[IBIS ver]   3.2
[File name]   sprm205b.ibs
[File Rev]   1.4
[Date]   Mar 27, 2006
[Disclaimer]   Please be aware that in the absence of a written agreement
|   Texas Instruments(TI) assumes no liability for:
|   (1) The accuracy of the IBIS models provided to your company
|   (2) The proper functioning of these Models in your design
|   or for any resulting applications
|   (3) Infringement of patents, copyrights or intellectual
|   property rights resulting from your use of these
|   models.
|   TI provides IBIS Models as a service to our customers and
|   therefore reserves the right to limit distribution of the
|   Models.
|   The information is subject to change without
|   notice.
[Copyright]   Property of Texas Instruments Incorporated.
|   Unauthorized reproduction and/or distribution is strictly.
|   prohibited.
|   This product is protected under copyright law and trade
|   secret law as an unpublished work.
|   Created 2003,(C) Copyright 1999-2003,
|   Texas Instruments Incorporated., All Rights Reserved.
|   These commodities are under the U.S. Government
|   distribution license control. As such,they are not to be
|   re-exported without the prior approval of the U.S.
|   Department of Commerce.
[Notes]
|   Some IV curves contain Non monotonic data
|   points.
|   Component C6455
[Component]   C6455
[Manufacturer]   Texas Instruments.
[Package]
| variable   typ   min   max
R_pkg   5.92E-01   2.06E-01   1.13E+00
L_pkg   2.81E-09   3.46E-10   4.56E-09
C_pkg   1.31E-12   8.61E-13   2.06E-12
[Pin]   signal_name   model_name   R_pin   L_pin   C_pin
AG4   VTXD3/FSX1/GP[11] BT3350DTHYPDFZSCP18   6.09E-01   2.80E-09   1.37E-12
AE5   VTXD2/FSR1/GP[10] BT3350DTHYPDFZSCP18   7.48E-01   2.34E-09   1.40E-12
AG5   VTXD1/DX1/GP[9]   BT3350DTHYPDFZSCP18   8.37E-01   2.90E-09   1.51E-12
AH5   VTXD0/DR1/GP[8]   BT3350DTHYPDFZSCP18   5.24E-01   3.12E-09   1.35E-12
AG6   VSCRUNz/CLKX0   BT3325ETHYPUFZSCP18   6.27E-01   2.86E-09   1.41E-12
AJ3   VRXD3/FSX0   BT3350DTHYPDFZSCP18   5.12E-01   3.46E-09   1.32E-12
AH3   VRXD2/FSR0   BT3350DTHYPDFZSCP18   8.46E-01   3.26E-09   1.65E-12
AF6   VRXD1/DX0   BT3350DTHYPDFZSCP18   7.73E-01   2.43E-09   1.47E-12
AJ5   VRXD0/DR0   BT3350DTHYPDFZSCP18   7.02E-01   3.32E-09   1.12E-12
AG1   VCLK/CLKR0   BT3325ETHYPUFZSCP18   5.49E-01   3.71E-09   1.40E-12
K3   UXSOC/MCOL/GMCOL  BT3350CTHYPDFZP18   3.31E-01   2.22E-09   1.04E-12
J5   UXENBz/MTXEN/RMTXEN BT3350CTHYPUFZP18   4.33E-01   1.80E-09   1.10E-12
N5   UXDATA7/GMTXD7   BT3350CTHYPUFZP18   4.15E-01   1.72E-09   1.08E-12
M3   UXDATA6/GMTXD6   BT3350CTHYPUFZP18   6.89E-01   2.16E-09   1.45E-12
L5   UXDATA5/GMTXD5   BT3350CTHYPUFZP18   6.34E-01   1.81E-09   1.41E-12
L3   UXDATA4/GMTXD4   BT3350CTHYPUFZP18   4.95E-01   2.20E-09   1.22E-12
K4   UXDATA3/MTXD3/GMTXD3 BT3350CTHYPUFZP18  6.82E-01   2.13E-09   1.38E-12
M4   UXDATA2/MTXD2/GMTXD2 BT3350CTHYPUFZP18  4.56E-01   1.96E-09   1.11E-12
L4   UXDATA1/MTXD1/RMTXD1 BT3350CTHYPUFZP18  2.86E-01   1.93E-09   1.06E-12
M1   UXDATA0/MTXD0/RMTXD0 BT3350CTHYPUFZP18  5.78E-01   2.81E-09   1.38E-12
N4   UXCLK/MTCLK/REFCLK BT3350DTHYPUFZSCP18  2.83E-01   1.84E-09   9.18E-13
K5   UXCLAV/GMTCLK   BT3350DTHYPDFZSCP18   4.28E-01   1.79E-09   1.14E-12
M5   UXADDR4/GMDCLK   BT3350CTHYPUFZP18   2.46E-01   1.67E-09   9.84E-13
N3   UXADDR3/GMDIO   BT3350CTHYPUFZP18   6.98E-01   2.32E-09   1.47E-12
P5   UXADDR2/PCBE3z   BPCI66RCGPUFZP18   4.09E-01   1.70E-09   1.09E-12
R3   UXADDR1/PIDSEL   BPCI66RCGPUFZP18   3.11E-01   2.12E-09   1.04E-12
P4   UXADDR0/PTRDYz   BPCI66RCGPUFZP18   6.39E-01   1.91E-09   1.40E-12
H4   URSOC/MRXER/RMRXER   BT3350CTHYPUFZP18  2.98E-01   1.99E-09   1.07E-12
H5   URENBz/MRXDV   BT3350CTHYPUFZP18   6.52E-01   1.96E-09   1.34E-12
M2   URDATA7/MRXD7   BT3350CTHYPUFZP18   3.58E-01   2.56E-09   1.02E-12
H2   URDATA6/MRXD6   BT3350CTHYPUFZP18   7.86E-01   2.83E-09   1.52E-12
L2   URDATA5/MRXD5   BT3350CTHYPUFZP18   7.58E-01   2.79E-09   1.61E-12
L1   URDATA4/MRXD4   BT3350CTHYPUFZP18   5.76E-01   2.73E-09   1.37E-12
J3   URDATA3/MRXD3   BT3350CTHYPUFZP18   5.17E-01   2.35E-09   1.24E-12
J1   URDATA2/MRXD2   BT3350CTHYPUFZP18   4.37E-01   2.85E-09   1.35E-12
H3   URDATA1/MRXD1/RMRXD1 BT3350CTHYPUFZP18  5.29E-01   2.45E-09   1.32E-12
J2   URDATA0/MRXD0/RMRXD0 BT3350CTHYPUFZP18  7.85E-01   2.80E-09   1.57E-12
H1   URCLK/MRCLK/GMRCLK   BT3350CTHYPUFZP18  4.59E-01   3.04E-09   1.26E-12
J4   URCLAV/MCRS/RMCRSDV  BT3350CTHYPDFZP18  6.78E-01   2.16E-09   1.45E-12
P1   URADDR4/PCBE0z/GP[2] BPCI66RCGPUFZP18   7.61E-01   2.71E-09   1.51E-12
P2   URADDR3/PREQz/GP[15] BPCI66RCGPUFZP18   5.35E-01   2.52E-09   1.27E-12
P3   URADDR2/PINTAz/GP14  BPCI66RCGPUFZP18   3.31E-01   2.20E-09   1.08E-12
R5   URADDR1/PRSTz/GP[13] BPCI66RCGPUFZP18   2.21E-01   1.50E-09   9.28E-13
R4   URADDR0/PGNTz/GP[12] BPCI66RCGPUFZP18   6.52E-01   1.98E-09   1.31E-12
AH7   TRST   IT33THYPDFZP18   4.68E-01   2.81E-09   1.20E-12
AG7   TOUTL1   BT3350CTHYPDFZP18   8.09E-01   2.65E-09   1.68E-12
AF8   TOUTL0   BT3350CTHYPDFZP18   7.76E-01   2.33E-09   1.43E-12
AJ10   TMS   IT33THYPUFZP18   8.57E-01   2.81E-09   1.63E-12
AJ6   TINPL1   BT3350CTHYPDFZP18   4.92E-01   2.86E-09   1.02E-12
AH6   TINPL0   BT3350CTHYPDFZP18   8.68E-01   3.06E-09   1.72E-12
AH8   TDO   BT3350DTHYPUFZSCP18   5.88E-01   2.38E-09   1.08E-12
AH9   TDI   IT33THYPUFZP18   6.08E-01   2.69E-09   1.30E-12
AJ9   TCK   IT33THYPUFZP18   8.56E-01   3.03E-09   1.59E-12
AJ13   SYSCLK3/GP[1]   BT3325ETHYPDFZSCP18   6.03E-01   2.77E-09   1.32E-12
AF26   SDA   BI2CTFZP18   8.57E-01   3.03E-09   1.71E-12
AG26   SCL   BI2CTFZP18   6.79E-01   3.07E-09   1.37E-12
AF15   RIOCLK   ICLKRX18G   5.07E-01   2.13E-09   1.25E-12
AG15   RIOCLKz   ICLKRX18G   7.35E-01   2.18E-09   1.43E-12
D3   RGTXCTL   BHSTLDVG   8.45E-01   2.76E-09   1.50E-12
D4   RGMTCLK   BHSTLDVG   6.15E-01   2.80E-09   1.29E-12
A2   RGMTD3   BHSTLDVG   5.94E-01   3.66E-09   1.40E-12
C3   RGMTD2   BHSTLDVG   8.89E-01   3.06E-09   1.64E-12
B3   RGMTD1   BHSTLDVG   9.28E-01   3.30E-09   1.78E-12
A3   RGMTD0   BHSTLDVG   7.46E-01   3.55E-09   1.43E-12
C2   RGMRXCTL   BHSTLDVG   4.83E-01   3.03E-09   1.27E-12
E3   RGMRCLK   BHSTLDVG   7.50E-01   2.59E-09   1.49E-12
C1   RGMRXD3   BHSTLDVG   8.67E-01   3.27E-09   1.63E-12
E4   RGMRXD2   BHSTLDVG   5.25E-01   2.45E-09   1.28E-12
E2   RGMRXD1   BHSTLDVG   4.36E-01   2.95E-09   1.29E-12
E1   RGMRXD0   BHSTLDVG   6.31E-01   3.09E-09   1.10E-12
A4   RGMDIO   BHSTLDVG   7.36E-01   3.49E-09   1.07E-12
B4   RGMDCLK   BHSTLDVG   9.25E-01   3.27E-09   1.59E-12
C4   RGREFCLK   BHSTLDVG   4.98E-01   2.98E-09   1.20E-12
AG14   RESETz   IT33THYP18   5.06E-01   2.06E-09   1.15E-12
AE14   RESETSTATz   BT3350CTHYPUFZP18   6.38E-01   1.67E-09   1.31E-12
Y29   PCI_EN   BT3350CTHYPDFZP18   9.60E-01   3.24E-09   1.91E-12
AH4   NMI   BT3350CTHYPDFZP18   9.04E-01   3.32E-09   1.67E-12
T5   HRWz/PCBE2z   BPCI66RCGPUFZP18   2.43E-01   1.60E-09   1.01E-12
T4   HRDYz/PIRDYz   BPCI66RCGPUFZP18   6.49E-01   2.01E-09   1.30E-12
U3   HINTz/PFRAMEz   BPCI66RCGPUFZP18   3.23E-01   2.16E-09   1.14E-12
V3   HHWIL/PCLK   BPCI66RCGPUFZP18   5.12E-01   2.31E-09   1.28E-12
U1   HDS2z/PCBE1z   BPCI66RCGPUFZP18   5.78E-01   2.75E-09   1.14E-12
U2   HDS1z/PSERRz   BPCI66RCGPUFZP18   7.38E-01   2.52E-09   1.46E-12
AA3   HD31/AD31   BPCI66RCGPUFZP18   3.58E-01   2.34E-09   1.14E-12
AA5   HD30/AD30   BPCI66RCGPUFZP18   6.55E-01   2.01E-09   1.37E-12
AC4   HD29/AD29   BPCI66RCGPUFZP18   3.31E-01   2.22E-09   1.11E-12
AA4   HD28/AD28   BPCI66RCGPUFZP18   4.88E-01   2.19E-09   1.08E-12
AC5   HD27/AD27   BPCI66RCGPUFZP18   6.86E-01   2.25E-09   1.38E-12
Y1   HD26/AD26   BPCI66RCGPUFZP18   4.37E-01   2.86E-09   1.30E-12
AD2   HD25/AD25   BPCI66RCGPUFZP18   6.04E-01   2.89E-09   1.50E-12
W1   HD24/AD24   BPCI66RCGPUFZP18   8.01E-01   2.91E-09   1.55E-12
AC3   HD23/AD23   BPCI66RCGPUFZP18   7.58E-01   2.69E-09   1.33E-12
AE1   HD22/AD22   BPCI66RCGPUFZP18   6.55E-01   3.17E-09   1.58E-12
AD1   HD21/AD21   BPCI66RCGPUFZP18   4.66E-01   3.11E-09   1.31E-12
W2   HD20/AD20   BPCI66RCGPUFZP18   3.62E-01   2.14E-09   1.16E-12
AC1   HD19/AD19   BPCI66RCGPUFZP18   8.42E-01   3.24E-09   1.66E-12
Y2   HD18/AD18   BPCI66RCGPUFZP18   5.80E-01   2.76E-09   1.37E-12
AB1   HD17/AD17   BPCI66RCGPUFZP18   4.42E-01   2.91E-09   1.42E-12
Y3   HD16/AD16   BPCI66RCGPUFZP18   7.19E-01   2.42E-09   1.39E-12
AB2   HD15/AD15   BPCI66RCGPUFZP18   5.75E-01   2.77E-09   1.38E-12
W4   HD14/AD14   BPCI66RCGPUFZP18   6.64E-01   2.06E-09   1.39E-12
AC2   HD13/AD13   BPCI66RCGPUFZP18   6.09E-01   2.99E-09   1.42E-12
V4   HD12/AD12   BPCI66RCGPUFZP18   6.63E-01   2.02E-09   1.46E-12
AF3   HD11/AD11   BPCI66RCGPUFZP18   8.21E-01   2.98E-09   1.63E-12
AE3   HD10/AD10   BPCI66RCGPUFZP18   5.92E-01   2.89E-09   1.46E-12
AB3   HD9/AD9   BPCI66RCGPUFZP18   7.51E-01   2.70E-09   1.51E-12
W5   HD8/AD8   BPCI66RCGPUFZP18   2.56E-01   1.70E-09   1.02E-12
AB4   HD7/AD7   BPCI66RCGPUFZP18   3.35E-01   2.26E-09   1.15E-12
Y4   HD6/AD6   BPCI66RCGPUFZP18   4.92E-01   2.22E-09   1.27E-12
AD3   HD5/AD5   BPCI66RCGPUFZP18   7.69E-01   2.75E-09   1.55E-12
Y5   HD4/AD4   BPCI66RCGPUFZP18   6.44E-01   1.93E-09   1.34E-12
AD4   HD3/AD3   BPCI66RCGPUFZP18   3.57E-01   2.45E-09   1.10E-12
W6   HD2/AD2   BPCI66RCGPUFZP18   5.81E-01   1.49E-09   1.29E-12
AB5   HD1/AD1   BPCI66RCGPUFZP18   4.60E-01   1.99E-09   1.21E-12
AE2   HD0/AD0   BPCI66RCGPUFZP18   8.34E-01   3.24E-09   1.63E-12
U6   HCSz/PPERRz   BPCI66RCGPUFZP18   2.06E-01   1.34E-09   8.91E-13
U4   HCNTL1/PDEVSELz   BPCI66RCGPUFZP18   4.64E-01   1.99E-09   1.20E-12
U5   HCNTL0/PSTOPz   BPCI66RCGPUFZP18   6.24E-01   1.79E-09   1.35E-12
T3   HASz/PPAR   BPCI66RCGPUFZP18   4.95E-01   2.25E-09   1.27E-12
AG2   GP[7]   BT3350DTHYPDFZSCP18   6.54E-01   3.32E-09   1.22E-12
AG3   GP[6]   BT3350DTHYPDFZSCP18   8.29E-01   3.14E-09   1.54E-12
AJ2   GP[5]   BT3350DTHYPDFZSCP18   7.00E-01   3.62E-09   1.55E-12
AH2   GP[4]   BT3350DTHYPDFZSCP18   5.15E-01   3.56E-09   1.32E-12
AE11   EMU1   BT3325ETHYPUFZSCP18   6.49E-01   1.74E-09   1.42E-12
AF7   EMU0   BT3325ETHYPUFZSCP18   5.81E-01   2.43E-09   1.23E-12
AE13   EMU18   BT3325ETHYPUFZSCP18   4.33E-01   1.56E-09   1.08E-12
AH10   EMU17   BT3325ETHYPUFZSCP18   5.89E-01   2.53E-09   1.32E-12
AE9   EMU15   BT3325ETHYPUFZSCP18   4.89E-01   1.94E-09   1.19E-12
AF13   EMU14   BT3325ETHYPUFZSCP18   7.13E-01   1.94E-09   1.31E-12
AD8   EMU13   BT3325ETHYPUFZSCP18   4.61E-01   1.70E-09   1.10E-12
AE10   EMU12   BT3325ETHYPUFZSCP18   4.69E-01   1.70E-09   1.11E-12
AH12   EMU16   BT3325ETHYPUFZSCP18   5.85E-01   2.50E-09   1.36E-12
AD12   EMU11   BT3325ETHYPUFZSCP18   4.10E-01   1.36E-09   1.01E-12
AD10   EMU10   BT3325ETHYPUFZSCP18   2.51E-01   1.42E-09   9.05E-13
AH13   EMU9   BT3325ETHYPUFZSCP18   3.95E-01   2.43E-09   1.19E-12
AF11   EMU8   BT3325ETHYPUFZSCP18   3.39E-01   1.96E-09   1.03E-12
AF12   EMU7   BT3325ETHYPUFZSCP18   3.19E-01   1.85E-09   9.89E-13
AG8   EMU6   BT3325ETHYPUFZSCP18   4.29E-01   2.55E-09   1.09E-12
AE12   EMU5   BT3325ETHYPUFZSCP18   6.73E-01   1.73E-09   1.31E-12
AF9   EMU4   BT3325ETHYPUFZSCP18   7.37E-01   2.16E-09   1.61E-12
AF10   EMU3   BT3325ETHYPUFZSCP18   7.24E-01   2.11E-09   1.43E-12
AG9   EMU2   BT3325ETHYPUFZSCP18   3.93E-01   2.36E-09   1.04E-12
AF5   CLKX1/GP[3]   BT3325ETHYPDFZSCP18   5.75E-01   2.45E-09   1.30E-12
AJ4   CLKS   BT3350CTHYPDFZP18   5.43E-01   3.41E-09   1.28E-12
AF4   CLKR1/GP[0]   BT3325ETHYPDFZSCP18   4.15E-01   2.53E-09   1.08E-12
G3   CLKIN2   IT33THYPDFZP18   5.43E-01   2.57E-09   9.68E-13
N28   CLKIN1   IT33THYPDFZP18   6.35E-01   2.69E-09   1.38E-12
B13   DSDWEz   BSSTL18GFZ   3.59E-01   2.46E-09   1.18E-12
C13   DSDRASz   BSSTL18GFZ   4.96E-01   2.18E-09   1.09E-12
E23   DSDDQS3   BSSTL18GFZ   3.31E-01   2.14E-09   1.04E-12
D23   DSDDQS3z   BSSTL18GFZ   5.26E-01   2.40E-09   1.19E-12
E20   DSDDQS2   BSSTL18GFZ   7.19E-01   2.12E-09   1.35E-12
D20   DSDDQS2z   BSSTL18GFZ   3.16E-01   2.01E-09   1.08E-12
E8   DSDDQS1   BSSTL18GFZ   5.55E-01   2.46E-09   1.20E-12
D8   DSDDQS1z   BSSTL18GFZ   3.91E-01   2.40E-09   1.08E-12
E11   DSDDQS0   BSSTL18GFZ   7.21E-01   2.10E-09   1.34E-12
D11   DSDDQS0z   BSSTL18GFZ   4.92E-01   2.23E-09   1.16E-12
C23   DSDDQM3   BSSTL18GFZ   7.78E-01   2.61E-09   1.47E-12
C20   DSDDQM2   BSSTL18GFZ   5.24E-01   2.35E-09   1.04E-12
C8   DSDDQM1   BSSTL18GFZ   8.23E-01   2.75E-09   1.58E-12
C11   DSDDQM0   BSSTL18GFZ   3.52E-01   2.28E-09   1.06E-12
F21   DSDDQGATE3   BSSTL18GFZ   2.22E-01   1.50E-09   1.03E-12
E21   DSDDQGATE2   BSSTL18GFZ   4.37E-01   1.80E-09   1.15E-12
B9   DSDDQGATE1   BSSTL18GFZ   5.56E-01   2.53E-09   1.09E-12
A9   DSDDQGATE0   BSSTL18GFZ   4.51E-01   3.00E-09   1.23E-12
D14   DSDCKE   BSSTL18GFZ   4.41E-01   1.88E-09   9.67E-13
D13   DSDCASz   BSSTL18GFZ   7.00E-01   2.09E-09   1.52E-12
A17   DEODT[1]   BSSTL18GFZ   5.57E-01   2.63E-09   1.08E-12
E16   DEODT[0]   BSSTL18GFZ   6.32E-01   1.50E-09   1.27E-12
B25   DED31   BSSTL18GFZ   6.19E-01   3.04E-09   1.50E-12
A25   DED30   BSSTL18GFZ   8.99E-01   3.42E-09   1.78E-12
B24   DED29   BSSTL18GFZ   6.02E-01   2.96E-09   1.33E-12
A24   DED28   BSSTL18GFZ   8.38E-01   2.95E-09   1.53E-12
D22   DED27   BSSTL18GFZ   2.92E-01   1.85E-09   1.07E-12
C22   DED26   BSSTL18GFZ   9.49E-01   2.59E-09   1.69E-12
B22   DED25   BSSTL18GFZ   5.68E-01   2.69E-09   1.45E-12
A22   DED24   BSSTL18GFZ   8.07E-01   2.44E-09   1.71E-12
D21   DED23   BSSTL18GFZ   7.04E-01   2.05E-09   1.47E-12
C21   DED22   BSSTL18GFZ   3.65E-01   2.38E-09   1.11E-12
B21   DED21   BSSTL18GFZ   9.23E-01   2.25E-09   1.74E-12
A21   DED20   BSSTL18GFZ   5.99E-01   2.82E-09   1.20E-12
D19   DED19   BSSTL18GFZ   7.00E-01   2.12E-09   1.47E-12
C19   DED18   BSSTL18GFZ   3.37E-01   2.21E-09   1.08E-12
A19   DED17   BSSTL18GFZ   9.35E-01   2.18E-09   1.76E-12
B19   DED16   BSSTL18GFZ   5.41E-01   2.48E-09   1.28E-12
C7   DED15   BSSTL18GFZ   5.66E-01   2.55E-09   1.33E-12
D7   DED14   BSSTL18GFZ   9.91E-01   2.78E-09   1.63E-12
A7   DED13   BSSTL18GFZ   4.73E-01   2.84E-09   1.29E-12
B7   DED12   BSSTL18GFZ   8.82E-01   3.15E-09   1.65E-12
F9   DED11   BSSTL18GFZ   4.47E-01   1.90E-09   1.15E-12
E9   DED10   BSSTL18GFZ   8.86E-01   2.18E-09   1.59E-12
D9   DED9   BSSTL18GFZ   3.32E-01   2.16E-09   9.59E-13
C9   DED8   BSSTL18GFZ   7.83E-01   2.64E-09   1.58E-12
D10   DED7   BSSTL18GFZ   7.11E-01   2.12E-09   1.47E-12
C10   DED6   BSSTL18GFZ   5.45E-01   2.29E-09   1.06E-12
B10   DED5   BSSTL18GFZ   9.48E-01   2.75E-09   1.69E-12
A10   DED4   BSSTL18GFZ   4.37E-01   2.82E-09   1.29E-12
D12   DED3   BSSTL18GFZ   6.89E-01   1.97E-09   1.40E-12
C12   DED2   BSSTL18GFZ   4.96E-01   2.18E-09   1.06E-12
B12   DED1   BSSTL18GFZ   7.89E-01   2.63E-09   1.57E-12
A12   DED0   BSSTL18GFZ   5.97E-01   2.80E-09   1.17E-12
B14   DDR2CLKOUTP   BSSTL18GFZ   8.23E-01   2.80E-09   1.52E-12
A14   DDR2CLKOUTN   BSSTL18GFZ   6.03E-01   2.82E-09   1.06E-12
B15   DEA13   BSSTL18GFZ   7.58E-01   2.40E-09   1.58E-12
A15   DEA12   BSSTL18GFZ   5.68E-01   2.69E-09   1.35E-12
A16   DEA11   BSSTL18GFZ   3.85E-01   2.51E-09   1.15E-12
B16   DEA10   BSSTL18GFZ   7.91E-01   2.45E-09   1.44E-12
C16   DEA9   BSSTL18GFZ   4.86E-01   2.11E-09   1.36E-12
D16   DEA8   BSSTL18GFZ   2.77E-01   1.84E-09   1.12E-12
B17   DEA7   BSSTL18GFZ   3.56E-01   2.32E-09   1.18E-12
C17   DEA6   BSSTL18GFZ   7.14E-01   2.33E-09   1.47E-12
D17   DEA5   BSSTL18GFZ   4.44E-01   1.89E-09   1.13E-12
E17   DEA4   BSSTL18GFZ   6.41E-01   1.65E-09   1.36E-12
A18   DEA3   BSSTL18GFZ   5.60E-01   2.58E-09   1.19E-12
B18   DEA2   BSSTL18GFZ   3.73E-01   2.45E-09   1.02E-12
C18   DEA1   BSSTL18GFZ   7.36E-01   2.41E-09   1.39E-12
D18   DEA0   BSSTL18GFZ   4.52E-01   1.89E-09   1.19E-12
E14   DCE0z   BSSTL18GFZ   6.49E-01   1.70E-09   1.23E-12
E15   DBA2   BSSTL18GFZ   2.38E-01   1.52E-09   9.14E-13
D15   DBA1   BSSTL18GFZ   6.83E-01   1.93E-09   1.44E-12
C15   DBA0   BSSTL18GFZ   4.95E-01   2.23E-09   1.11E-12
AB25   AAWEz/ASWEz   BT3350DTHYPUFZSCP18   7.69E-01   1.99E-09   1.65E-12
W25   AR/Wz   BT3350DTHYPUFZSCP18   3.14E-01   1.65E-09   9.87E-13
Y28   AAOEz/ASOEz   BT3350DTHYPUFZSCP18   8.31E-01   2.20E-09   1.72E-12
R29   AHOLDz   BT3350CTHYPUFZP18   9.46E-01   3.13E-09   1.81E-12
N26   AHOLDAz   BT3350CTHYPUFZP18   5.24E-01   2.00E-09   1.23E-12
F25   AED63   BT3350DTHYPUFZSCP18   7.89E-01   2.15E-09   1.36E-12
A27   AED62   BT3350DTHYPUFZSCP18   7.72E-01   3.71E-09   1.62E-12
C27   AED61   BT3350DTHYPUFZSCP18   9.51E-01   3.23E-09   1.70E-12
C28   AED60   BT3350DTHYPUFZSCP18   7.67E-01   3.66E-09   1.45E-12
E27   AED59   BT3350DTHYPUFZSCP18   4.68E-01   2.81E-09   1.26E-12
D28   AED58   BT3350DTHYPUFZSCP18   9.58E-01   3.21E-09   1.69E-12
D27   AED57   BT3350DTHYPUFZSCP18   6.67E-01   2.99E-09   1.30E-12
F27   AED56   BT3350DTHYPUFZSCP18   6.45E-01   2.81E-09   1.25E-12
G25   AED55   BT3350DTHYPUFZSCP18   5.37E-01   2.10E-09   1.23E-12
G26   AED54   BT3350DTHYPUFZSCP18   4.19E-01   2.36E-09   1.16E-12
A28   AED53   BT3350DTHYPUFZSCP18   6.54E-01   3.93E-09   1.43E-12
F28   AED52   BT3350DTHYPUFZSCP18   9.26E-01   3.02E-09   2.03E-12
B28   AED51   BT3350DTHYPUFZSCP18   1.04E+00   3.74E-09   1.95E-12
G27   AED50   BT3350DTHYPUFZSCP18   6.38E-01   2.73E-09   1.34E-12
B27   AED49   BT3350DTHYPUFZSCP18   5.58E-01   3.17E-09   1.43E-12
G28   AED48   BT3350DTHYPUFZSCP18   4.85E-01   2.82E-09   1.19E-12
H25   AED47   BT3350DTHYPUFZSCP18   7.81E-01   2.11E-09   1.46E-12
J26   AED46   BT3350DTHYPUFZSCP18   8.14E-01   2.33E-09   1.57E-12
H26   AED45   BT3350DTHYPUFZSCP18   5.78E-01   2.36E-09   9.76E-13
J27   AED44   BT3350DTHYPUFZSCP18   5.96E-01   2.46E-09   1.32E-12
H27   AED43   BT3350DTHYPUFZSCP18   4.51E-01   2.58E-09   1.04E-12
J28   AED42   BT3350DTHYPUFZSCP18   4.69E-01   2.75E-09   1.22E-12
C29   AED41   BT3350DTHYPUFZSCP18   1.13E+00   4.35E-09   2.00E-12
J29   AED40   BT3350DTHYPUFZSCP18   9.53E-01   3.20E-09   1.86E-12
D29   AED39   BT3350DTHYPUFZSCP18   8.22E-01   3.89E-09   1.64E-12
J25   AED38   BT3350DTHYPUFZSCP18   3.47E-01   1.87E-09   9.91E-13
F29   AED37   BT3350DTHYPUFZSCP18   1.02E+00   3.63E-09   1.81E-12
F26   AED36   BT3350DTHYPUFZSCP18   8.37E-01   2.44E-09   1.66E-12
G29   AED35   BT3350DTHYPUFZSCP18   7.03E-01   3.11E-09   1.43E-12
K28   AED34   BT3350DTHYPUFZSCP18   5.98E-01   2.38E-09   1.45E-12
K25   AED33   BT3350DTHYPUFZSCP18   4.94E-01   1.76E-09   1.18E-12
K27   AED32   BT3350DTHYPUFZSCP18   8.53E-01   2.56E-09   1.72E-12
AA27   AED31   BT3350DTHYPUFZSCP18   5.91E-01   2.40E-09   1.33E-12
AG29   AED30   BT3350DTHYPUFZSCP18   7.73E-01   3.53E-09   1.63E-12
AB29   AED29   BT3350DTHYPUFZSCP18   7.00E-01   3.16E-09   1.20E-12
AC27   AED28   BT3350DTHYPUFZSCP18   4.26E-01   2.49E-09   1.13E-12
AB28   AED27   BT3350DTHYPUFZSCP18   4.67E-01   2.64E-09   1.12E-12
AC26   AED26   BT3350DTHYPUFZSCP18   8.05E-01   2.21E-09   1.60E-12
AB27   AED25   BT3350DTHYPUFZSCP18   8.55E-01   2.52E-09   1.64E-12
AC25   AED24   BT3350DTHYPUFZSCP18   5.12E-01   1.92E-09   1.15E-12
AB26   AED23   BT3350DTHYPUFZSCP18   5.46E-01   2.14E-09   1.28E-12
AD28   AED22   BT3350DTHYPUFZSCP18   4.68E-01   2.73E-09   1.08E-12
AD29   AED21   BT3350DTHYPUFZSCP18   9.46E-01   3.09E-09   1.86E-12
AJ28   AED20   BT3350DTHYPUFZSCP18   1.03E+00   4.07E-09   1.99E-12
AF29   AED19   BT3350DTHYPUFZSCP18   5.92E-01   3.44E-09   1.38E-12
AH28   AED18   BT3350DTHYPUFZSCP18   7.85E-01   3.68E-09   1.24E-12
AE29   AED17   BT3350DTHYPUFZSCP18   7.43E-01   3.46E-09   1.30E-12
AG28   AED16   BT3350DTHYPUFZSCP18   1.01E+00   3.59E-09   1.91E-12
AF28   AED15   BT3350DTHYPUFZSCP18   7.10E-01   3.12E-09   1.36E-12
AH26   AED14   BT3350DTHYPUFZSCP18   5.35E-01   3.16E-09   1.25E-12
AE28   AED13   BT3350DTHYPUFZSCP18   9.42E-01   3.10E-09   1.71E-12
AE26   AED12   BT3350DTHYPUFZSCP18   8.60E-01   3.00E-09   1.59E-12
AD26   AED11   BT3350DTHYPUFZSCP18   3.97E-01   2.39E-09   1.10E-12
AF27   AED10   BT3350DTHYPUFZSCP18   5.31E-01   3.20E-09   1.14E-12
AG27   AED9   BT3350DTHYPUFZSCP18   9.16E-01   3.29E-09   1.87E-12
AD27   AED8   BT3350DTHYPUFZSCP18   5.75E-01   2.48E-09   1.27E-12
AE25   AED7   BT3350DTHYPUFZSCP18   5.96E-01   2.68E-09   1.20E-12
AJ27   AED6   BT3350DTHYPUFZSCP18   6.28E-01   3.87E-09   1.50E-12
AJ26   AED5   BT3350DTHYPUFZSCP18   9.46E-01   3.47E-09   1.88E-12
AE27   AED4   BT3350DTHYPUFZSCP18   6.54E-01   3.06E-09   1.02E-12
AG25   AED3   BT3350DTHYPUFZSCP18   4.92E-01   3.03E-09   1.26E-12
AH27   AED2   BT3350DTHYPUFZSCP18   7.32E-01   3.30E-09   1.46E-12
AF25   AED1   BT3350DTHYPUFZSCP18   6.26E-01   2.91E-09   1.20E-12
AD25   AED0   BT3350DTHYPUFZSCP18   7.53E-01   2.34E-09   1.47E-12
V29   AECLKOUT   BT3325ETHYPDFZSCP18   9.72E-01   3.21E-09   2.06E-12
N29   AECLKIN   BT3350CTHYPDFZP18   9.47E-01   3.14E-09   1.80E-12
T26   AEA2/CFGGP2   BT3350DTHYPDFZSCP18   5.04E-01   1.89E-09   1.17E-12
N25   AEA19/BOOTMODE3   BT3350DTHYPDFZSCP18   3.15E-01   1.66E-09   9.71E-13
L26   AEA18/BOOTMODE2   BT3350DTHYPDFZSCP18   5.31E-01   2.00E-09   1.31E-12
L25   AEA17/BOOTMODE1   BT3350DTHYPDFZSCP18   7.40E-01   1.80E-09   1.58E-12
P26   AEA16/BOOTMODE0   BT3350DTHYPDFZSCP18   5.34E-01   2.05E-09   1.34E-12
P27   AEA15/AECLKIN_SEL BT3350DTHYPDFZSCP18   4.13E-01   2.30E-09   1.12E-12
R25   AEA14/HPI_WIDTH   BT3350DTHYPDFZSCP18   4.42E-01   1.39E-09   1.14E-12
R27   AEA13/LENDIAN   BT3350DTHYPDFZSCP18   3.97E-01   2.24E-09   1.17E-12
R28   AEA12/UTOPIA_EN   BT3350DTHYPDFZSCP18   8.31E-01   2.41E-09   1.73E-12
T25   AEA11   BT3350DTHYPDFZSCP18   3.16E-01   1.69E-09   9.17E-13
M25   AEA10/MACSEL1   BT3350DTHYPDFZSCP18   7.26E-01   1.71E-09   1.54E-12
U26   AEA1/CFGGP1   BT3350DTHYPDFZSCP18   3.66E-01   2.03E-09   1.05E-12
M27   AEA9/MACSEL0   BT3350DTHYPDFZSCP18   4.25E-01   2.38E-09   1.05E-12
P25   AEA8/PCI_EEAI   BT3350DTHYPDFZSCP18   3.02E-01   1.61E-09   9.65E-13
N27   AEA7/VLYNQ_EN   BT3350DTHYPDFZSCP18   5.39E-01   2.15E-09   1.34E-12
U27   AEA6/PCI66   BT3350DTHYPDFZSCP18   7.77E-01   2.14E-09   1.62E-12
U28   AEA5/MCBSP1_EN   BT3350DTHYPDFZSCP18   4.30E-01   2.43E-09   8.61E-13
T28   AEA4/SYSCLKOUT_EN BT3350DTHYPDFZSCP18   5.99E-01   2.52E-09   1.38E-12
T27   AEA3   BT3350DTHYPDFZSCP18   7.71E-01   2.11E-09   1.61E-12
U25   AEA0/CFGGP0   BT3350DTHYPDFZSCP18   4.70E-01   1.62E-09   1.15E-12
V27   ACE5z   BT3350DTHYPUFZSCP18   3.83E-01   2.13E-09   1.01E-12
V28   ACE4z   BT3350DTHYPUFZSCP18   5.91E-01   2.56E-09   1.27E-12
W26   ACE3z   BT3350DTHYPUFZSCP18   5.27E-01   2.06E-09   1.24E-12
W27   ACE2z   BT3350DTHYPUFZSCP18   8.17E-01   2.36E-09   1.61E-12
L27   ABUSREQ   BT3350DTHYPUFZSCP18   4.02E-01   2.29E-09   1.05E-12
W29   ABE7z   BT3350DTHYPUFZSCP18   1.03E+00   3.63E-09   2.03E-12
K26   ABE6z   BT3350DTHYPUFZSCP18   3.76E-01   2.10E-09   1.10E-12
L29   ABE5z   BT3350DTHYPUFZSCP18   9.16E-01   2.89E-09   1.91E-12
L28   ABE4z   BT3350DTHYPUFZSCP18   6.07E-01   2.47E-09   1.36E-12
AA29   ABE3z   BT3350DTHYPUFZSCP18   4.82E-01   2.72E-09   1.27E-12
AA28   ABE2z   BT3350DTHYPUFZSCP18   8.84E-01   2.66E-09   1.70E-12
AA25   ABE1z   BT3350DTHYPUFZSCP18   7.53E-01   1.85E-09   1.54E-12
AA26   ABE0z   BT3350DTHYPUFZSCP18   3.69E-01   2.09E-09   1.05E-12
V25   ABA1/EMIFA_EN   BT3350DTHYPDFZSCP18   4.77E-01   1.65E-09   1.13E-12
V26   ABA0/DDR2_EN   BT3350DTHYPDFZSCP18   7.70E-01   2.05E-09   1.58E-12
K29   AARDY   BT3350CTHYPUFZP18   9.29E-01   3.07E-09   1.75E-12
R26   ASADS/ASRE   BT3350DTHYPUFZSCP18   5.17E-01   1.94E-09   1.32E-12
| Reserved Pins
|N1 		Reserved
|V5 		Reserved
|W3 		Reserved
|N11		Reserved
|P11		Reserved
|L6 		Reserved
|G4 		Reserved
|F3 		Reserved
|D26 		Reserved
|A26 		Reserved
|D24		Reserved
|C24		Reserved
|F2 		Reserved
|F1 		Reserved
|T1 		Reserved
|T2 		Reserved
|AE21 		Reserved
|E13 		Reserved
|F18 		Reserved
|U29 		Reserved
|A6 		Reserved
|B26 		Reserved
|C26 		Reserved
|B6 		Reserved
|C6 		Reserved
|AJ11 		Reserved
|AH11 		Reserved
|N7 		Reserved
|N6 		Reserved
|P23 		Reserved
|D25 		Reserved
|C25 		Reserved
|E6 		Reserved
|D6 		Reserved
|AD11 		Reserved
|AD9 		Reserved
|AG10 		Reserved
|AG11 		Reserved
|AJ12 		Reserved
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[Diff Pin]   inv_pin  vdiff   tdelay_typ
AF15   AG15   250mV   NA
[Model Selector]   BT3350DTHYPUFZSCP18
BT3350DTHYPUFZSCP180 50 ohm impedance with "fastest" slew rate.
[Model Selector]   BT3350DTHYPDFZSCP18
BT3350DTHYPDFZSCP180  50 ohm impedance with "fastest" slew rate.
[Model Selector]   BT3325ETHYPUFZSCP18
BT3325ETHYPUFZSCP180 50 ohm impedance with "fastest" slew rate.
[Model Selector]   BT3325ETHYPDFZSCP18
BT3325ETHYPDFZSCP180 50 ohm impedance with "fastest" slew rate.
[Model Selector]   BHSTLDVG
BHSTLDVG_1.5V_00   50 ohm impedance with "fastest" slew rate.
BHSTLDVG_1.8V_00   50 ohm impedance with "fastest" slew rate.
[Model Selector]   BSSTL18GFZ
BSSTL18GFZ_Z50_SR11   50 ohm impedance with "slowest" slew rate.
| Models and submodels in the file (15): BT3350CTHYPUFZP18 (I/O), BT3350CTHYPDFZP18 (I/O), BT3350DTHYPUFZSCP180 (I/O), BT3350DTHYPDFZSCP180 (I/O), BT3325ETHYPUFZSCP180 (I/O), BT3325ETHYPDFZSCP180 (I/O), BPCI66RCGPUFZP18 (I/O), IT33THYPUFZP18 (Input), IT33THYPDFZP18 (Input), BI2CTFZP18 (I/O_open_drain), ICLKRX18G (Input), BHSTLDVG_1.5V_00 (I/O), BHSTLDVG_1.8V_00 (I/O), BSSTL18GFZ_Z50_SR11 (I/O), IT33THYP18 (Input)
